ORGANIZATION_BLOCK OB 1
BEGIN

	// Check instance-DB length
	AUF		DB 1
	L		DBLG
	__ASSERT==	__ACCU 1,	22
	AUF		DB 0


	// Check TP pulse
	CALL	SFB 3, DB 1 (
		IN	:= FALSE,
		PT	:= T#0S,
		Q	:= M 0.0,
		ET	:= MD 2,
	)
	U		M 0.0
	__ASSERT==	__STW VKE,	0
	L		MD 2
	__ASSERT==	__ACCU 1,	0
	L		DB1.DBB 12	// STATE
	__ASSERT==	__ACCU 1,	0
	L		DB1.DBD 14	// STIME
	__ASSERT==	__ACCU 1,	0
	L		DB1.DBD 18	// ATIME
	__ASSERT>=	__ACCU 1,	__ACCU 2

	CALL	SFB 3, DB 1 (
		IN	:= FALSE,
		PT	:= T#100MS,
		Q	:= M 0.0,
		ET	:= MD 2,
	)
	U		M 0.0
	__ASSERT==	__STW VKE,	0
	L		MD 2
	__ASSERT==	__ACCU 1,	0
	L		DB1.DBB 12	// STATE
	__ASSERT==	__ACCU 1,	0
	L		DB1.DBD 14	// STIME
	__ASSERT==	__ACCU 1,	0
	L		DB1.DBD 18	// ATIME
	__ASSERT>=	__ACCU 1,	__ACCU 2

	CALL	SFB 3, DB 1 (
		IN	:= TRUE,
		PT	:= T#100MS,
		Q	:= M 0.0,
		ET	:= MD 2,
	)
	U		M 0.0
	__ASSERT==	__STW VKE,	1
	L		MD 2
	__ASSERT>=	__ACCU 1,	0
	L		DB1.DBB 12	// STATE
	__ASSERT==	__ACCU 1,	1
	L		DB1.DBD 14	// STIME
	__ASSERT<>	__ACCU 1,	0
	L		DB1.DBD 18	// ATIME
	__ASSERT>=	__ACCU 1,	__ACCU 2

	__SLEEP		90
	CALL	SFB 3, DB 1 (
		IN	:= TRUE,
		PT	:= T#100MS,
		Q	:= M 0.0,
		ET	:= MD 2,
	)
	U		M 0.0
	__ASSERT==	__STW VKE,	1
	L		MD 2
	__ASSERT>	__ACCU 1,	80
	__ASSERT<	__ACCU 1,	100
	L		DB1.DBB 12	// STATE
	__ASSERT==	__ACCU 1,	1
	L		DB1.DBD 14	// STIME
	__ASSERT<>	__ACCU 1,	0
	L		DB1.DBD 18	// ATIME
	__ASSERT>=	__ACCU 1,	__ACCU 2

	__SLEEP		11
	CALL	SFB 3, DB 1 (
		IN	:= TRUE,
		PT	:= T#100MS,
		Q	:= M 0.0,
		ET	:= MD 2,
	)
	U		M 0.0
	__ASSERT==	__STW VKE,	0
	L		MD 2
	__ASSERT==	__ACCU 1,	100
	L		DB1.DBB 12	// STATE
	__ASSERT==	__ACCU 1,	2
	L		DB1.DBD 14	// STIME
	__ASSERT<>	__ACCU 1,	0
	L		DB1.DBD 18	// ATIME
	__ASSERT>=	__ACCU 1,	__ACCU 2

	CALL	SFB 3, DB 1 (
		IN	:= FALSE,
		PT	:= T#100MS,
		Q	:= M 0.0,
		ET	:= MD 2,
	)
	U		M 0.0
	__ASSERT==	__STW VKE,	0
	L		MD 2
	__ASSERT==	__ACCU 1,	0
	L		DB1.DBB 12	// STATE
	__ASSERT==	__ACCU 1,	0
	L		DB1.DBD 14	// STIME
	__ASSERT<>	__ACCU 1,	0
	L		DB1.DBD 18	// ATIME
	__ASSERT>=	__ACCU 1,	__ACCU 2


	// Test: Interrupt IN before time elapsed
	CALL	SFB 3, DB 1 (
		IN	:= TRUE,
		PT	:= T#100MS,
		Q	:= M 0.0,
		ET	:= MD 2,
	)
	U		M 0.0
	__ASSERT==	__STW VKE,	1
	L		MD 2
	__ASSERT>=	__ACCU 1,	0
	L		DB1.DBB 12	// STATE
	__ASSERT==	__ACCU 1,	1
	L		DB1.DBD 14	// STIME
	__ASSERT<>	__ACCU 1,	0
	L		DB1.DBD 18	// ATIME
	__ASSERT>=	__ACCU 1,	__ACCU 2

	__SLEEP		40
	CALL	SFB 3, DB 1 (
		IN	:= TRUE,
		PT	:= T#100MS,
		Q	:= M 0.0,
		ET	:= MD 2,
	)
	U		M 0.0
	__ASSERT==	__STW VKE,	1
	L		MD 2
	__ASSERT>	__ACCU 1,	30
	__ASSERT<	__ACCU 1,	50
	L		DB1.DBB 12	// STATE
	__ASSERT==	__ACCU 1,	1
	L		DB1.DBD 14	// STIME
	__ASSERT<>	__ACCU 1,	0
	L		DB1.DBD 18	// ATIME
	__ASSERT>=	__ACCU 1,	__ACCU 2

	__SLEEP		40
	CALL	SFB 3, DB 1 (
		IN	:= FALSE,
		PT	:= T#100MS,
		Q	:= M 0.0,
		ET	:= MD 2,
	)
	U		M 0.0
	__ASSERT==	__STW VKE,	1
	L		MD 2
	__ASSERT>	__ACCU 1,	70
	__ASSERT<	__ACCU 1,	90
	L		DB1.DBB 12	// STATE
	__ASSERT==	__ACCU 1,	1
	L		DB1.DBD 14	// STIME
	__ASSERT<>	__ACCU 1,	0
	L		DB1.DBD 18	// ATIME
	__ASSERT>=	__ACCU 1,	__ACCU 2

	__SLEEP		21
	CALL	SFB 3, DB 1 (
		IN	:= FALSE,
		PT	:= T#100MS,
		Q	:= M 0.0,
		ET	:= MD 2,
	)
	U		M 0.0
	__ASSERT==	__STW VKE,	0
	L		MD 2
	__ASSERT==	__ACCU 1,	0
	L		DB1.DBB 12	// STATE
	__ASSERT==	__ACCU 1,	0
	L		DB1.DBD 14	// STIME
	__ASSERT<>	__ACCU 1,	0
	L		DB1.DBD 18	// ATIME
	__ASSERT>=	__ACCU 1,	__ACCU 2


	// Test: Change PT while running
	CALL	SFB 3, DB 1 (
		IN	:= TRUE,
		PT	:= T#100MS,
		Q	:= M 0.0,
		ET	:= MD 2,
	)
	U		M 0.0
	__ASSERT==	__STW VKE,	1
	L		MD 2
	__ASSERT>=	__ACCU 1,	0
	L		DB1.DBB 12	// STATE
	__ASSERT==	__ACCU 1,	1
	L		DB1.DBD 14	// STIME
	__ASSERT<>	__ACCU 1,	0
	L		DB1.DBD 18	// ATIME
	__ASSERT>=	__ACCU 1,	__ACCU 2

	__SLEEP		40
	CALL	SFB 3, DB 1 (
		IN	:= TRUE,
		PT	:= T#100MS,
		Q	:= M 0.0,
		ET	:= MD 2,
	)
	U		M 0.0
	__ASSERT==	__STW VKE,	1
	L		MD 2
	__ASSERT>	__ACCU 1,	30
	__ASSERT<	__ACCU 1,	50
	L		DB1.DBB 12	// STATE
	__ASSERT==	__ACCU 1,	1
	L		DB1.DBD 14	// STIME
	__ASSERT<>	__ACCU 1,	0
	L		DB1.DBD 18	// ATIME
	__ASSERT>=	__ACCU 1,	__ACCU 2

	CALL	SFB 3, DB 1 (
		IN	:= TRUE,
		PT	:= T#0MS,
		Q	:= M 0.0,
		ET	:= MD 2,
	)
	U		M 0.0
	__ASSERT==	__STW VKE,	0
	L		MD 2
	__ASSERT==	__ACCU 1,	0
	L		DB1.DBB 12	// STATE
	__ASSERT==	__ACCU 1,	0
	L		DB1.DBD 14	// STIME
	__ASSERT<>	__ACCU 1,	0
	L		DB1.DBD 18	// ATIME
	__ASSERT>=	__ACCU 1,	__ACCU 2

	CALL	SFB 3, DB 1 (
		IN	:= FALSE,
		PT	:= T#0MS,
		Q	:= M 0.0,
		ET	:= MD 2,
	)
	U		M 0.0
	__ASSERT==	__STW VKE,	0
	L		MD 2
	__ASSERT==	__ACCU 1,	0
	L		DB1.DBB 12	// STATE
	__ASSERT==	__ACCU 1,	0
	L		DB1.DBD 14	// STIME
	__ASSERT<>	__ACCU 1,	0
	L		DB1.DBD 18	// ATIME
	__ASSERT>=	__ACCU 1,	__ACCU 2


	// Test: At PT=0 the timer is not started
	CALL	SFB 3, DB 1 (
		IN	:= TRUE,
		PT	:= T#0MS,
		Q	:= M 0.0,
		ET	:= MD 2,
	)
	U		M 0.0
	__ASSERT==	__STW VKE,	0
	L		MD 2
	__ASSERT==	__ACCU 1,	0
	L		DB1.DBB 12	// STATE
	__ASSERT==	__ACCU 1,	0
	L		DB1.DBD 14	// STIME
	__ASSERT<>	__ACCU 1,	0
	L		DB1.DBD 18	// ATIME
	__ASSERT>=	__ACCU 1,	__ACCU 2
	U		DB1.DBX 0.0	// IN
	__ASSERT==	__STW VKE,	0	// IN will be forced low.

	CALL	SFB 3, DB 1 (
		IN	:= FALSE,
		PT	:= T#0MS,
		Q	:= M 0.0,
		ET	:= MD 2,
	)
	U		M 0.0
	__ASSERT==	__STW VKE,	0
	L		MD 2
	__ASSERT==	__ACCU 1,	0
	L		DB1.DBB 12	// STATE
	__ASSERT==	__ACCU 1,	0
	L		DB1.DBD 14	// STIME
	__ASSERT<>	__ACCU 1,	0
	L		DB1.DBD 18	// ATIME
	__ASSERT>=	__ACCU 1,	__ACCU 2
	U		DB1.DBX 0.0	// IN
	__ASSERT==	__STW VKE,	0


	CALL SFC 46 // STOP CPU
END_ORGANIZATION_BLOCK


DATA_BLOCK DB 1
	SFB 3
BEGIN
END_DATA_BLOCK
